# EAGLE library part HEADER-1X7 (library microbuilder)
PIN HEADER
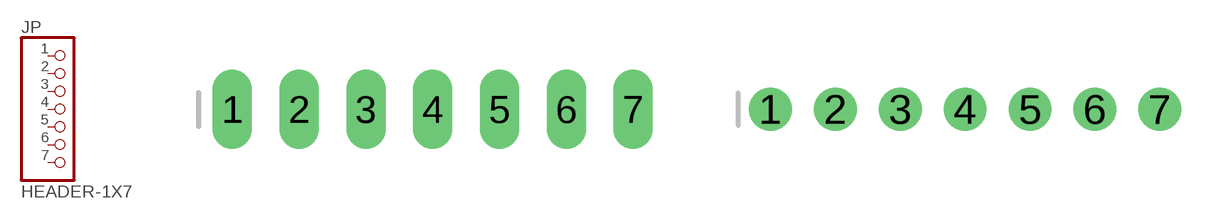
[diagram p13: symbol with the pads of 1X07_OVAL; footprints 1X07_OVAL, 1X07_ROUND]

Designator prefix JP

## HEADER-1X7  [1X07_OVAL]
1  1  pas
2  2  pas
3  3  pas
4  4  pas
5  5  pas
6  6  pas
7  7  pas

## HEADER-1X7ROUND  [1X07_ROUND]
Pads as for 1X07_OVAL

## HEADER-1X7THICKER  [1X07_ROUND_76]
Pads as for 1X07_OVAL

## HEADER-1X770MIL  [1X07_ROUND_70]
Pads as for 1X07_OVAL

## Footprint 1X07_OVAL (pad centres in mm)
PIN HEADER
drill 1 long: 1 -7.62,0; 2 -5.08,0; 3 -2.54,0; 4 0,0; 5 2.54,0; 6 5.08,0; 7 7.62,0

## Footprint 1X07_ROUND (pad centres in mm)
drill 1 pad 1.676: 1 -7.62,0; 2 -5.08,0; 3 -2.54,0; 4 0,0; 5 2.54,0; 6 5.08,0; 7 7.62,0

## Footprint 1X07_ROUND_76 (pad centres in mm)
drill 1 pad 1.93: 1 -7.62,0; 2 -5.08,0; 3 -2.54,0; 4 0,0; 5 2.54,0; 6 5.08,0; 7 7.62,0

## Footprint 1X07_ROUND_70 (pad centres in mm)
drill 1 pad 1.778: 1 -7.62,0; 2 -5.08,0; 3 -2.54,0; 4 0,0; 5 2.54,0; 6 5.08,0; 7 7.62,0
